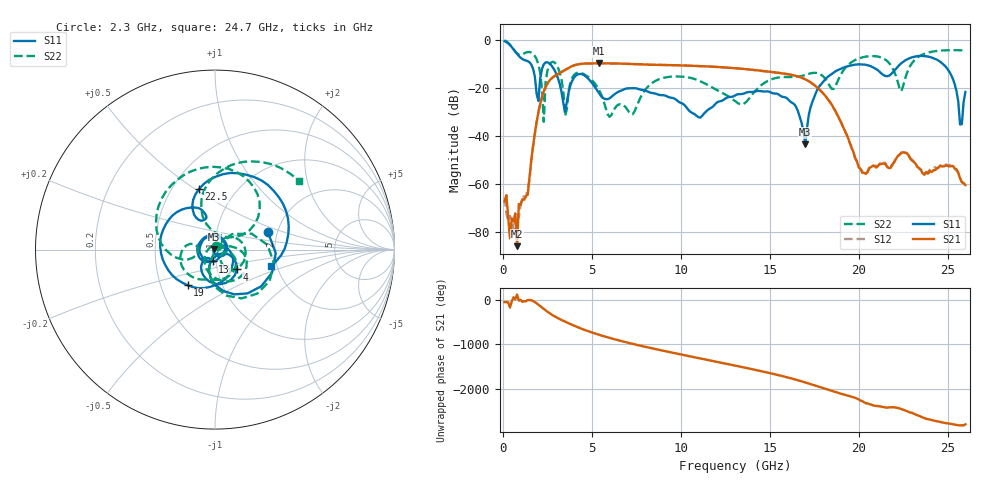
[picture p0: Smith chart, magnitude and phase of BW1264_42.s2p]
!Keysight Technologies,N5245B,MY57181159,A.13.60.06
!Date: Friday, December 18, 2020 23:54:19
!Correction: S11(Full 2 Port(1,2))
!S21(Full 2 Port(1,2))
!S12(Full 2 Port(1,2))
!S22(Full 2 Port(1,2))
!S2P File: Measurements: S11, S21, S12, S22:
# Hz S  dB  R 50
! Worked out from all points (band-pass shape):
!   260 points, 100 MHz to 26 GHz, reference 50 ohm
!   highest |S21| = -9.74 dB at 5.4 GHz (marker M1); lowest = -86.1 dB at 800 MHz (marker M2)
!   |S21| within 3 dB of the highest: 3.445 GHz to 14.4 GHz (10.95 GHz wide, 123 % of centre)
!   lowest |S11| = -43.6 dB at 17 GHz (marker M3), VSWR 1.01, Z = 49.5 + j0.384 ohm
!   |S11| at or under -10 dB: 1.575 GHz to 2.323 GHz (748.2 MHz wide, 38.4 % of centre); 2.65 GHz to 22.35 GHz (19.7 GHz wide, 158 % of centre); 24.73 GHz to end of sweep
!   |S22| runs from -34.2 to -0.2 dB; largest |S21 - S12| = 0.00063
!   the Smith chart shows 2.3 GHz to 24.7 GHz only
!   S11 on the Smith chart (normalised r, x): 2.3 GHz: 1.78, +0.38; 4 GHz: 1.24, -0.28; 13 GHz: 0.97, -0.13; 19 GHz: 0.69, -0.29; 22.5 GHz: 0.68, +0.52; 24.7 GHz: 1.85, -0.38
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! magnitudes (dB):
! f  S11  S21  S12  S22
! 100 MHz  -0.5  -67.4  -66.0  -0.2
! 800 MHz  -5.8  -86.1  -72.1  -5.7
! 1.9 GHz  -22.5  -34.2  -34.3  -8.1
! 2.3 GHz  -10.2  -21.5  -21.5  -34.2
! 2.7 GHz  -10.3  -16.3  -16.3  -9.5
! 3.5 GHz  -29.9  -12.5  -12.5  -31.7
! 4 GHz  -15.7  -10.6  -10.6  -14.6
! 4.5 GHz  -14.4  -9.9  -9.9  -14.1
! 5.4 GHz  -22.2  -9.7  -9.7  -20.8
! 7.3 GHz  -20.2  -10.1  -10.1  -31.0
! 8.8 GHz  -22.9  -10.4  -10.4  -16.3
! 13 GHz  -23.4  -11.7  -11.8  -25.2
! 13.1 GHz  -23.0  -11.8  -11.8  -25.7
! 16 GHz  -24.5  -14.2  -14.2  -15.4
! 17 GHz  -43.6  -16.4  -16.4  -14.6
! 17.4 GHz  -25.7  -18.2  -18.2  -13.8
! 19 GHz  -12.0  -34.2  -34.2  -14.4
! 21.7 GHz  -14.9  -53.5  -53.6  -9.5
! 22.5 GHz  -9.1  -46.9  -46.7  -19.3
! 24.7 GHz  -9.8  -52.8  -52.3  -4.4
! 25.7 GHz  -35.3  -57.7  -57.6  -4.3
! 26 GHz  -21.7  -60.5  -61.5  -4.3
